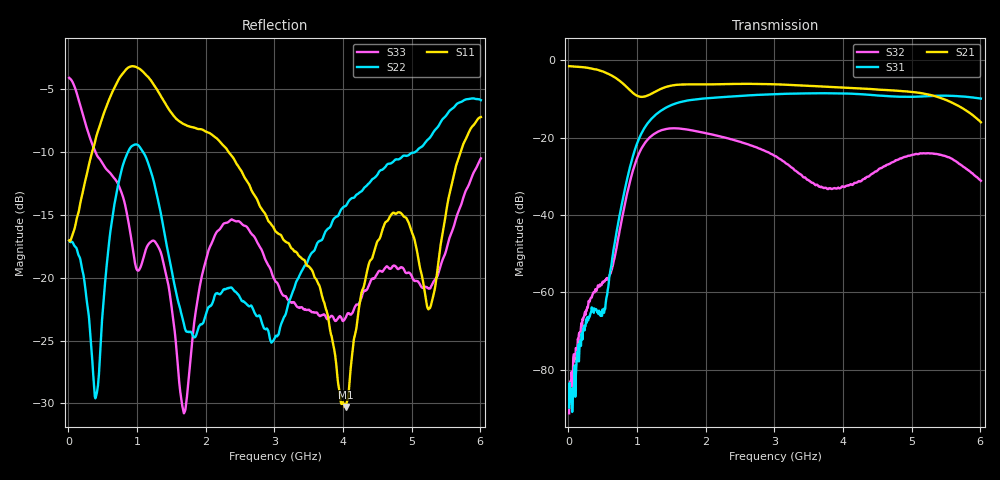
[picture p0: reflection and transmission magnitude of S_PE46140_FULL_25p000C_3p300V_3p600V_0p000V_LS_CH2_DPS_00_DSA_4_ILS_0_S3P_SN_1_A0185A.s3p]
! Device ID: PE46140_FULL
! File Path: z:\PE46140\MajorStates\25p000C\3p300\LS_CH2_DPS_00_DSA_4_ILS_0\PE46140_FULL_25p000C_3p300V_3p600V_0p000V_LS_CH2_DPS_00_DSA_4_ILS_0_S3P_SN_1_A0185A.s3p
! Serial: 1
! Lot: A0185A
! Temp: 25.000C
! VDD: 3.300
! VSS: 0.000
! Control_Hi: 3.600
! Control_Lo: 0.000
! Logic State: LS_CH2_DPS_00_DSA_4_ILS_0
! Port 1: RFIN
! Port 2: RFOUT1
! Port 3: RFOUT2
! ThroughPath:1-3
! IDD: 0.0003148027
! ISS: -1.744e-007
! Comment:
#  Hz  S  RI  R  50
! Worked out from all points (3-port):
!   801 points, 10 MHz to 6.01 GHz, reference 50 ohm
!   strongest paths, dB at 10 MHz, 1.51 GHz, 3.01 GHz, 4.51 GHz, 6.01 GHz:
!     S21: -1.5, -6.5, -6.2, -7.6, -16.0
!     S31: -89.8, -11.5, -8.7, -9.1, -9.9
!     S32: -91.3, -17.6, -24.7, -28.4, -31.1
!   lowest |S11| = -30.3 dB at 4.037 GHz (marker M1), VSWR 1.06, Z = 47.2 + j1.03 ohm
!   |S11| at or under -10 dB: start of sweep to 346.1 MHz; 2.332 GHz to 5.716 GHz (3.385 GHz wide, 84.1 % of centre)
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1e7  0.1401 -0.0108  0.8421 -0.0245  3.22e-05 -6.67e-07
     0.8417 -0.0245  0.14 -0.00674  -3.53e-05 -1.36e-05
     2.97e-05 -1.27e-05  -2e-05 1.84e-05  0.6196 -0.0582
3.625e8  -0.0232 -0.3262  0.4449 -0.6345  -0.000532 -0.000257
         0.4457 -0.632  -0.0129 -0.0386  -7.84e-05 0.000926
         -0.000558 -0.000256  -8.09e-05 0.000986  -0.3007 -0.1381
1.165e9  -0.5849 0.2224  -0.2057 -0.2881  -0.1557 -0.0228
         -0.2059 -0.2886  0.2133 -0.1866  -0.00228 0.0966
         -0.1562 -0.0232  -0.00232 0.0967  0.1109 0.0781
1.6825e9  -0.2844 0.2914  -0.4885 -0.0223  0.1965 0.2211
          -0.4887 -0.0225  0.0339 -0.056  -0.00545 -0.129
          0.1968 0.2215  -0.00528 -0.1291  -0.0274 -0.00928
2.1625e9  -0.0992 0.3435  -0.3135 0.3771  0.2665 -0.1956
          -0.3138 0.3772  0.0773 -0.0392  -0.0875 0.0603
          0.2669 -0.1958  -0.0877 0.0605  0.1063 0.1087
3.01e9  0.0392 0.1488  0.4066 0.274  -0.316 -0.1847
        0.4062 0.2749  -0.0577 -0.00181  0.052 -0.0249
        -0.3166 -0.185  0.0522 -0.0252  0.0967 -0.0105
4.0375e9  -0.0286 0.0109  0.0425 -0.4411  -0.00915 0.3729
          0.0431 -0.4415  0.1395 0.1326  0.0192 0.0136
          -0.00811 0.3726  0.0192 0.0136  0.0687 0.00888
4.81e9  -0.1802 -0.0244  -0.4038 -0.00499  0.3336 0.062
        -0.4039 -0.00623  0.2941 0.0238  -0.0516 -0.00758
        0.3339 0.0616  -0.0518 -0.00712  0.1026 -0.0344
5.26e9  -0.0587 -0.0475  -0.1708 0.3159  0.288 -0.1905
        -0.1719 0.3159  0.3575 -0.0185  -0.00745 0.0625
        0.2882 -0.1904  -0.00709 0.0624  0.0905 0.00526
6.01e9  -0.3265 -0.2869  0.1509 0.0461  -0.1428 -0.2862
        0.1514 0.0465  0.2471 -0.4432  0.0249 -0.0123
        -0.1442 -0.2867  0.0247 -0.0125  0.2756 0.113
